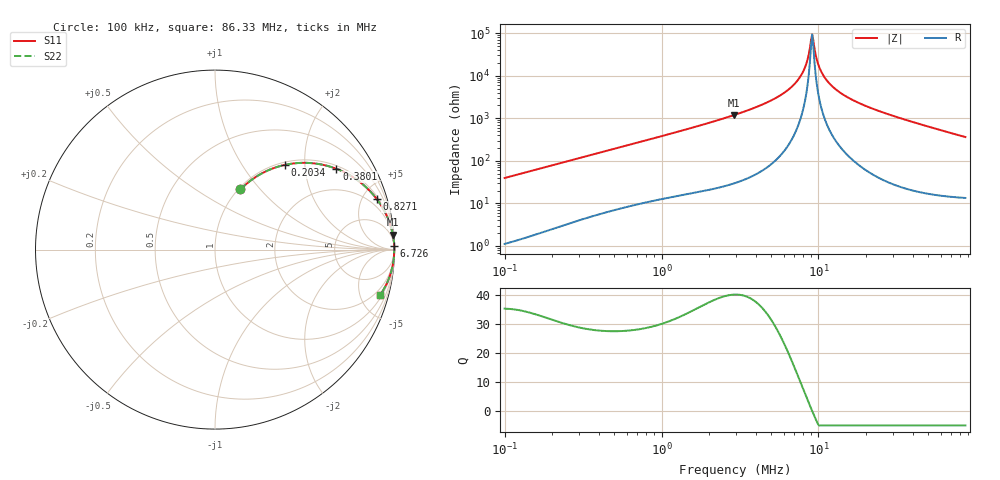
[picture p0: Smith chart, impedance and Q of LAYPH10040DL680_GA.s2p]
! LAYPH10040DL680_GA  S-PARAMETER MODEL  ( General Type )
! Model Generated by TAIYO YUDEN Corporation (http://www.ty-top.com)
! Version 1.0
! TAIYO YUDEN Control No. 180920NI43SB-FBB
! Copyright(c) 2018 TAIYO YUDEN CO.,LTD. All Rights Reserved.
! Product Description (link to TY-COMPAS)
! https://ds.yuden.co.jp/TYCOMPAS/or/detail?pn=LAYPH10040DL680MGA&u=M
! Products Name : Inductors
! Characteristics :
!  Inductance : 68 uH , SRF(min) : -Hz , DC Resistance(max) : 0.216 Ohm
!  Rated Current : Saturation :1.4 A , Temp Rise : 0.74 A (25 degC)
!  Case Size : 10.1 x 10.0 / 0.398 x 0.394 [mm/inch] , Thickness : 4 / 0.157 [mm/inch]
!  (Conditions: Temperature = 25 degC , DC Bias Current/Voltage = 0A / 0V)
! External Node Assignments :
!  1  o---GGG---o  2
! GND o---------o GND
! Frequency Range : 0.1MHz  -  86.325287MHz  [ 402 STEP ]
# MHz S RI R 50
! Freq[MHz].  S11 Real  S11 Imag  S21 Real  S21 Imag  S12 Real  S12 Imag  S22 Real  S22 Imag
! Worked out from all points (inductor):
!   401 points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, 100 kHz to 86.33 MHz, reference 50 ohm
!   read as one part in series: L = 62.6 uH near 103.4 kHz
!   highest Q = 40.3 at 2.889 MHz (marker M1), where L = 65.2 uH
!   self-resonance near 8.965 MHz
!   S11 on the Smith chart (normalised r, x): 100 kHz: 1.02, +0.79; 203.4 kHz: 1.05, +1.59; 380.1 kHz: 1.10, +2.93; 827.1 kHz: 1.22, +6.28; 6.726 MHz: open; 86.33 MHz: 1.27, -7.22
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0.1  0.1418 0.335  0.8582 -0.335  0.8582 -0.335  0.1418 0.335
0.203374  0.3906 0.4723  0.6094 -0.4723  0.6094 -0.4723  0.3906 0.4723
0.310315  0.588 0.4751  0.412 -0.4751  0.412 -0.4751  0.588 0.4751
0.380091  0.6764 0.4503  0.3236 -0.4503  0.3236 -0.4503  0.6764 0.4503
0.827072  0.9 0.2832  0.1 -0.2832  0.1 -0.2832  0.9 0.2832
0.962956  0.9231 0.2502  0.0769 -0.2502  0.0769 -0.2502  0.9231 0.2502
2.888874  0.9909 0.0835  0.00913 -0.0835  0.00913 -0.0835  0.9909 0.0835
2.938117  0.9912 0.0818  0.0088 -0.0818  0.0088 -0.0818  0.9912 0.0818
4.878422  0.9972 0.0396  0.0028 -0.0396  0.0028 -0.0396  0.9972 0.0396
6.725831  0.9986 0.0184  0.00138 -0.0184  0.00138 -0.0184  0.9986 0.0184
7.443685  0.9988 0.0121  0.00118 -0.0121  0.00118 -0.0121  0.9988 0.0121
7.964332  0.9989 0.00806  0.0011 -0.00806  0.0011 -0.00806  0.9989 0.00806
8.37858  0.9989 0.00502  0.00107 -0.00502  0.00107 -0.00502  0.9989 0.00502
8.964618  0.9989 0.000993  0.00107 -0.000993  0.00107 -0.000993  0.9989 0.000993
9.117424  0.9989 -1.09e-05  0.00107 1.09e-05  0.00107 1.09e-05  0.9989 -1.09e-05
9.272834  0.9989 -0.00101  0.00108 0.00101  0.00108 0.00101  0.9989 -0.00101
9.921421  0.9989 -0.00503  0.00114 0.00503  0.00114 0.00503  0.9989 -0.00503
10.43746  0.9988 -0.00805  0.00121 0.00805  0.00121 0.00805  0.9988 -0.00805
12.35943  0.9984 -0.0183  0.00159 0.0183  0.00159 0.0183  0.9984 -0.0183
17.03982  0.997 -0.0392  0.00301 0.0392  0.00301 0.0392  0.997 -0.0392
28.29276  0.9913 -0.0812  0.0087 0.0812  0.0087 0.0812  0.9913 -0.0812
86.32529  0.9209 -0.252  0.0791 0.252  0.0791 0.252  0.9209 -0.252
